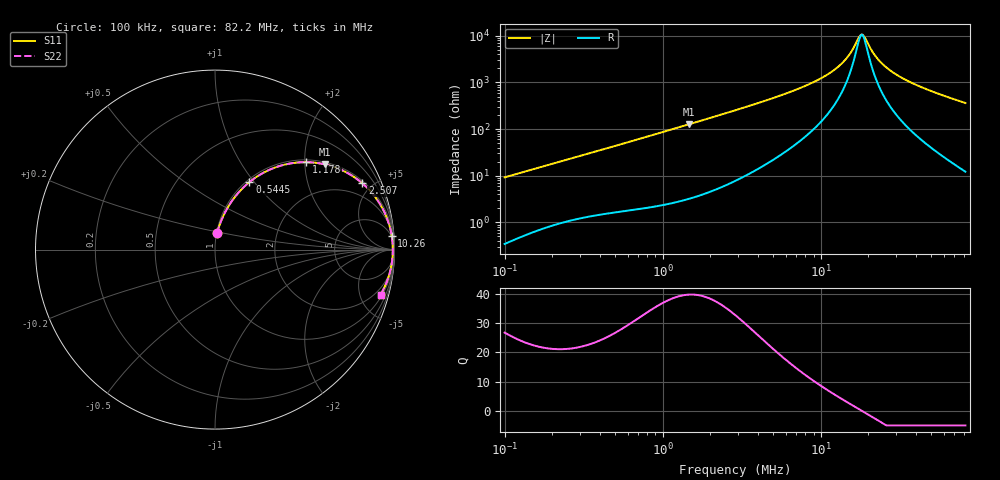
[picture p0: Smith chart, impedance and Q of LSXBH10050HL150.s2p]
! LSXBH10050HL150  S-PARAMETER MODEL  ( General Type )
! Model Generated by TAIYO YUDEN Corporation (http://www.ty-top.com)
! Version 3.0
! TAIYO YUDEN Control No. 180118NI43SB-FBB
! Copyright(c) 2007 TAIYO YUDEN CO.,LTD. All Rights Reserved.
! Product Description (link to TY-COMPAS)
! https://ds.yuden.co.jp/TYCOMPAS/or/detail?pn=LSXBH10050HL150M&u=M
! Products Name : Inductors
! Characteristics :
!  Inductance : 15 uH , SRF(min) : 11 MHz , DC Resistance(max) : 0.0455 Ohm
!  Rated Current : Saturation :3600 mA , Temp Rise : 3200 mA (40 degC)
!  Case Size : 10.0 x 9.8 / 0.394 x 0.386 [mm/inch] , Thickness : 5 / 0.197 [mm/inch]
!  (Conditions: Temperature = 25 degC , DC Bias Current/Voltage = 0A / 0V)
! External Node Assignments :
!  1  o---GGG---o  2
! GND o---------o GND
! Frequency Range : 0.1MHz  -  82.198079MHz  [ 402 STEP ]
# MHz S RI R 50
! Freq[MHz].  S11 Real  S11 Imag  S21 Real  S21 Imag  S12 Real  S12 Imag  S22 Real  S22 Imag
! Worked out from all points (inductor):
!   401 points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, 100 kHz to 82.2 MHz, reference 50 ohm
!   read as one part in series: L = 14.6 uH near 103.4 kHz
!   highest Q = 39.7 at 1.465 MHz (marker M1), where L = 13.8 uH
!   self-resonance near 18.16 MHz
!   S11 on the Smith chart (normalised r, x): 100 kHz: 1.01, +0.18; 544.5 kHz: 1.03, +0.95; 1.178 MHz: 1.05, +2.03; 2.507 MHz: 1.12, +4.38; 10.26 MHz: 4, +25; 82.2 MHz: 1.24, -7.25
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0.1  0.0118 0.0908  0.9882 -0.0908  0.9882 -0.0908  0.0118 0.0908
0.307779  0.0787 0.2474  0.9213 -0.2474  0.9213 -0.2474  0.0787 0.2474
0.544506  0.1915 0.3759  0.8085 -0.3759  0.8085 -0.3759  0.1915 0.3759
0.947281  0.4036 0.477  0.5964 -0.477  0.5964 -0.477  0.4036 0.477
1.17818  0.5084 0.4871  0.4916 -0.4871  0.4916 -0.4871  0.5084 0.4871
1.465361  0.6134 0.4745  0.3866 -0.4745  0.3866 -0.4745  0.6134 0.4745
2.50688  0.8208 0.3695  0.1792 -0.3695  0.1792 -0.3695  0.8208 0.3695
2.867021  0.8566 0.3355  0.1434 -0.3355  0.1434 -0.3355  0.8566 0.3355
5.424287  0.9542 0.185  0.0458 -0.185  0.0458 -0.185  0.9542 0.185
8.824095  0.9807 0.0982  0.0193 -0.0982  0.0193 -0.0982  0.9807 0.0982
10.26253  0.9848 0.0756  0.0152 -0.0756  0.0152 -0.0756  0.9848 0.0756
12.13741  0.9879 0.0522  0.0121 -0.0522  0.0121 -0.0522  0.9879 0.0522
13.88108  0.9895 0.0344  0.0105 -0.0344  0.0105 -0.0344  0.9895 0.0344
15.35134  0.9902 0.0215  0.00976 -0.0215  0.00976 -0.0215  0.9902 0.0215
17.55672  0.9907 0.00447  0.00929 -0.00447  0.00929 -0.00447  0.9907 0.00447
18.1559  0.9907 0.000248  0.00927 -0.000248  0.00927 -0.000248  0.9907 0.000248
19.09322  0.9907 -0.00609  0.0093 0.00609  0.0093 0.00609  0.9907 -0.00609
22.5814  0.99 -0.0274  0.01 0.0274  0.01 0.0274  0.99 -0.0274
27.15873  0.9881 -0.0517  0.0119 0.0517  0.0119 0.0517  0.9881 -0.0517
32.66391  0.9847 -0.0775  0.0153 0.0775  0.0153 0.0775  0.9847 -0.0775
42.01221  0.9769 -0.1164  0.0231 0.1164  0.0231 0.1164  0.9769 -0.1164
82.19808  0.9221 -0.2517  0.0779 0.2517  0.0779 0.2517  0.9221 -0.2517
